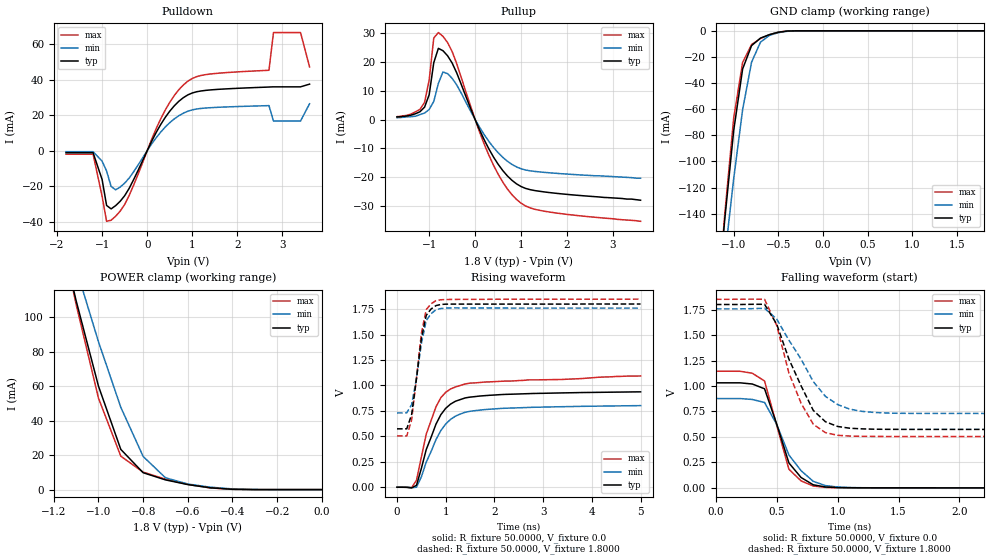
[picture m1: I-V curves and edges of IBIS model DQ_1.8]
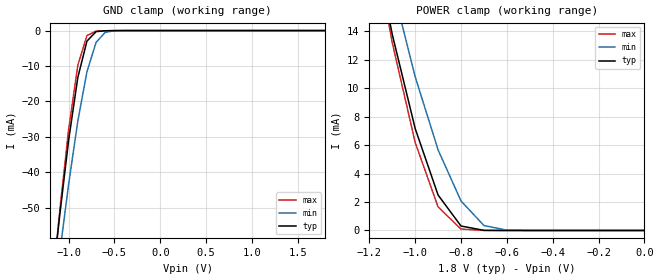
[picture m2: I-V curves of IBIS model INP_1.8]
|*** ISSI Synchronous Sram IBIS Model ***
[IBIS ver]	3.2
[File name]	is61vvps204836b119bg.ibs
[File Rev]	1.0
[Date]	May 13,2013
[Notes]
|--- Version History --------------------------------
|1.0: prelimiary
[Disclaimer]	This information is for modeling purpose only
		and is not guaranteed
[Copyright]	INTEGRATED SILICON SOLUTION, INC. 2011
[Component]	IS61VVPS204836B_119BGA
[Manufacturer]	ISSI
[Package]
| variable   typ   min   max
R_pkg		100.34m			23.84m			218.59m
L_pkg		1.3400nH		0.3700nH		3.0300nH
C_pkg		41.410pF		0.4200pF		150.38pF
[Pin]  signal_name   model_name   R_pin   L_pin   C_pin
U7   VDDQ   POWER
U6   NC   NC
U5   TDO   DQ_1.8
U4   TCK   INP_1.8
U3   TDI   INP_1.8
U2   TMS   INP_1.8
U1   VDDQ   POWER
T7   ZZ   INP_1.8
T6   A   INP_1.8
T5   A   INP_1.8
T4   A   INP_1.8
T3   A   INP_1.8
T2   A   INP_1.8
T1   NC   NC
R7   NC   NC
R6   A   INP_1.8
R5   NC   NC
R4   VDD   POWER
R3   MODE   INP_1.8
R2   A   INP_1.8
R1   NC   NC
P7   DQa   DQ_1.8
P6   DQPa   DQ_1.8
P5   VSS   GND
P4   A0   INP_1.8
P3   VSS   GND
P2   DQPd   DQ_1.8
P1   DQd   DQ_1.8
N7   DQa   DQ_1.8
N6   DQa   DQ_1.8
N5   VSS   GND
N4   A1   INP_1.8
N3   VSS   GND
N2   DQd   DQ_1.8
N1   DQd   DQ_1.8
M7   VDDQ   POWER
M6   DQa   DQ_1.8
M5   VSS   GND
M4   BWEB   INP_1.8
M3   VSS   GND
M2   DQd   DQ_1.8
M1   VDDQ   POWER
L7   DQa   DQ_1.8
L6   DQa   DQ_1.8
L5   BWaB   INP_1.8
L4   NC   NC
L3   BWdB   INP_1.8
L2   DQd   DQ_1.8
L1   DQd   DQ_1.8
K7   DQa   DQ_1.8
K6   DQa   DQ_1.8
K5   VSS   GND
K4   CLK   INP_1.8
K3   VSS   GND
K2   DQd   DQ_1.8
K1   DQd   DQ_1.8
J7   VDDQ   POWER
J6   VDD   POWER
J5   NC   NC
J4   VDD   POWER
J3   NC   NC
J2   VDD   POWER
J1   VDDQ   POWER
H7   DQb   DQ_1.8
H6   DQb   DQ_1.8
H5   VSS   GND
H4   GWB   INP_1.8
H3   VSS   GND
H2   DQc   DQ_1.8
H1   DQc   DQ_1.8
G7   DQb   DQ_1.8
G6   DQb   DQ_1.8
G5   BWbB   INP_1.8
G4   ADVB   INP_1.8
G3   BWcB   INP_1.8
G2   DQc   DQ_1.8
G1   DQc   DQ_1.8
F7   VDDQ   POWER
F6   DQb   DQ_1.8
F5   VSS   GND
F4   OEB   INP_1.8
F3   VSS   GND
F2   DQc   DQ_1.8
F1   VDDQ   POWER
E7   DQb   DQ_1.8
E6   DQb   DQ_1.8
E5   VSS   GND
E4   CEB   INP_1.8
E3   VSS   GND
E2   DQc   DQ_1.8
E1   DQc   DQ_1.8
D7   DQb   DQ_1.8
D6   DQPb   DQ_1.8
D5   VSS   GND
D4   NC   NC
D3   VSS   GND
D2   DQPc   DQ_1.8
D1   DQc   DQ_1.8
C7   NC   Nc
C6   A   INP_1.8
C5   A   INP_1.8
C4   VDD   POWER
C3   A   INP_1.8
C2   A   INP_1.8
C1   NC   NC
B7   NC   NC
B6   A   INP_1.8
B5   A   INP_1.8
B4   ADSCB   INP_1.8
B3   A   INP_1.8
B2   A   INP_1.8
B1   NC   NC
A7   VDDQ   POWER
A6   A   INP_1.8
A5   A   INP_1.8
A4   ADSPB   INP_1.8
A3   A   INP_1.8
A2   A   INP_1.8
A1   VDDQ   POWER
| Models and submodels in the file (2): DQ_1.8 (3-state), INP_1.8 (Input)
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|   Model DQ_1.8
[Model]		DQ_1.8
Model_type	3-state
Polarity   Non-Inverting
Enable   Active-Low
Vmeas = 	0.7500V
Cref = 		5.0000pF
Rref = 		50.0000
Vref = 		0.8000V
C_comp   3.8290pF   3.3420pF   4.0300pF|
[Temperature Range]	  25.0000   100.0000   0.0
[Voltage Range]   1.8000V   1.7000V   1.9000V
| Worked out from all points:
|   slope of the pulldown table from 0 to 0.27 V, typ, clamps not added: 20.1 ohm
|   slope of the pullup table from 0 to 0.27 V, typ, clamps not added: 29.1 ohm
|   GND clamp passes 1 mA (typ) near -0.49 V on its own axis
|   POWER clamp passes 1 mA (typ) near -0.49 V on its own axis
|   rising waveform, R_fixture 50.0000, V_fixture 0.0: 20-80 % time 458ps typ, 504ps min, 428ps max; typ from 0 V to 0.937 V
|   rising waveform, R_fixture 50.0000, V_fixture 1.8000: 20-80 % time 212ps typ, 215ps min, 202ps max; typ from 0.574 V to 1.8 V
|   falling waveform, R_fixture 50.0000, V_fixture 0.0: 20-80 % time 184ps typ, 232ps min, 159ps max; typ from 1.03 V to 0 V
|   falling waveform, R_fixture 50.0000, V_fixture 1.8000: 20-80 % time 261ps typ, 323ps min, 225ps max; typ from 1.8 V to 0.574 V
[Pulldown]
|Voltage	  I(typ)   I(min)   I(max)
-1.8V     -1.1mA     -531.4uA   -1.933mA
-1.2V     -1.1mA     -531.4uA   -1.933mA
-1V       -16.17mA   -5.85mA    -25.61mA
-900mV    -30.82mA   -11.44mA   -39.73mA
-800mV    -32.74mA   -20.11mA   -39.13mA
-400mV    -21.21mA   -15.41mA   -25.25mA
400mV     18.75mA    13.32mA    22.87mA
900mV     31.42mA    22.22mA    39.13mA
2.7V      35.87mA    25.41mA    45.31mA
2.8V      35.97mA    16.71mA    66.53mA
3.4V      35.97mA    16.71mA    66.53mA
3.6V      37.5mA     26.46mA    47.19mA
[Pullup]
|Voltage	  I(typ)   I(min)   I(max)
-1.7V     900uA      630uA      990uA
-1.3V     2mA        1.134mA    2.662mA
-1.1V     4.3mA      2.25mA     5.962mA
-1V       8.6mA      3.483mA    13.72mA
-900mV    19.73mA    6.273mA    28.28mA
-800mV    24.69mA    12.51mA    30.17mA
-700mV    23.88mA    16.48mA    28.87mA
-500mV    19.6mA     14.29mA    23.58mA
300mV     -10.22mA   -7.61mA    -12.41mA
900mV     -22.31mA   -16.43mA   -27.72mA
1.5V      -25.11mA   -18.32mA   -31.79mA
3.6V      -28mA      -20.34mA   -35.31mA
[GND_clamp]
|Voltage	  I(typ)   I(min)   I(max)
-1.8V     -699.5mA   -630.9mA   -769.6mA
-1.2V     -220.2mA   -237.3mA   -225.5mA
-1.1V     -144.4mA   -173.5mA   -140.5mA
-1V       -76.37mA   -113.2mA   -66.75mA
-900mV    -29.2mA    -60.35mA   -24.21mA
-800mV    -11.34mA   -23.99mA   -10.5mA
-700mV    -5.573mA   -8.7mA     -5.882mA
-600mV    -2.907mA   -3.456mA   -3.007mA
-500mV    -1.075mA   -1.407mA   -999.2uA
-400mV    -173.9uA   -365.4uA   -128uA
1.8V      2.34nA     184.5nA    2.08nA
[POWER_clamp]
|Voltage	  I(typ)   I(min)   I(max)
-1.8V     524.9mA    464.4mA    580.5mA
-1.2V     164.3mA    173.4mA    169.2mA
-1.1V     109.5mA    128.3mA    107.3mA
-1V       59.99mA    85.74mA    53.06mA
-900mV    23.31mA    47.72mA    19.37mA
-800mV    9.803mA    19.24mA    10.14mA
-700mV    5.64mA     6.854mA    6.056mA
-600mV    2.92mA     3.245mA    3.006mA
-500mV    1.061mA    1.426mA    981.4uA
-400mV    183.6uA    396.9uA    135.3uA
0V        2.34nA     17.95nA    3.205nA
[Ramp]
| variable   typ   min   max
dV/dt_r		0.5623/0.4256n   0.4811/0.4247n   0.6354/0.4100n
dV/dt_f		0.7357/0.2222n   0.6457/0.2069n   0.7931/0.2538n
R_load =	50.0000
[Rising Waveform]
R_fixture=	50.0000
V_fixture=	0.0
V_fixture_min=	0.0
V_fixture_max=	0.0
|time   V(typ)   V(min)   V(max)
0s        0V         0V         0V
300ps     -6.035mV   -4.762mV   -4.194mV
400ps     18.96mV    486.8uV    69.03mV
600ps     370.5mV    247mV      521.7mV
800ps     620mV      467.9mV    790.2mV
900ps     712.9mV    557.2mV    879.6mV
1.1ns     817.3mV    666.8mV    965.5mV
1.4ns     877.6mV    736.7mV    1.015V
1.9ns     903.3mV    766.6mV    1.035V
5ns       937.2mV    801.8mV    1.093V
[Rising Waveform]
R_fixture=	50.0000
V_fixture=	1.8000
V_fixture_min=	1.8500
V_fixture_max=	1.7500
|time   V(typ)   V(min)   V(max)
0s        573.8mV    730.3mV    504.1mV
200ps     573.9mV    730.3mV    504.2mV
300ps     713.7mV    812.3mV    659.4mV
400ps     1.067V     1.071V     1.076V
500ps     1.46V      1.412V     1.51V
600ps     1.689V     1.637V     1.745V
700ps     1.752V     1.705V     1.802V
800ps     1.784V     1.744V     1.833V
1.2ns     1.799V     1.762V     1.845V
5ns       1.8V       1.76V      1.848V
[Falling Waveform]
R_fixture=	50.0000
V_fixture=	0.0
V_fixture_min=	0.0
V_fixture_max=	0.0
|time   V(typ)   V(min)   V(max)
0s        1.031V     876.6mV    1.145V
300ps     1.019V     867.6mV    1.125V
400ps     972.5mV    838.1mV    1.049V
500ps     626.1mV    622.4mV    612.9mV
600ps     244.7mV    322.8mV    182.9mV
700ps     101.5mV    168.6mV    68.26mV
800ps     29.89mV    63.85mV    18.06mV
900ps     8.638mV    22.26mV    4.629mV
1.2ns     563.4uV    1.383mV    368.3uV
5ns       26.68uV    38.84uV    22.23uV
[Falling Waveform]
R_fixture=	50.0000
V_fixture=	1.8000
V_fixture_min=	1.8500
V_fixture_max=	1.7500
|time   V(typ)   V(min)   V(max)
0s        1.8V       1.757V     1.851V
400ps     1.802V     1.763V     1.851V
500ps     1.607V     1.657V     1.594V
600ps     1.264V     1.45V      1.127V
700ps     1.002V     1.263V     831.3mV
800ps     760.7mV    1.044V     624.3mV
900ps     649.1mV    898.2mV    542.1mV
1.1ns     585.4mV    772.7mV    508.4mV
1.4ns     574.7mV    734.9mV    504.6mV
5ns       573.8mV    730.3mV    504.2mV
|   Model INP_1.8
[Model]		INP_1.8
Model_type	Input
Polarity   Non-Inverting
Enable   Active-Low
Vinl = 		0.4000V
Vinh = 		1.6000V
C_comp   3.8290pF   3.3420pF   4.0300pF|
[Temperature Range]	  25.0000   100.0000   0.0
[Voltage Range]   1.8000V   1.7000V   1.9000V
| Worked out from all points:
|   GND clamp passes 1 mA (typ) near -0.73 V on its own axis
|   POWER clamp passes 1 mA (typ) near -0.83 V on its own axis
[GND_clamp]
|Voltage	  I(typ)   I(min)   I(max)
-1.8V     -237.3mA   -225.6mA   -256.2mA
-1.2V     -76.89mA   -84.89mA   -78.19mA
-1.1V     -52.83mA   -63.46mA   -51.66mA
-1V       -30.98mA   -43.42mA   -27.92mA
-900mV    -13.28mA   -25.61mA   -9.811mA
-800mV    -2.971mA   -11.61mA   -1.401mA
-700mV    -287uA     -3.303mA   -148.3uA
-600mV    -52.18uA   -480.7uA   -48.72uA
-500mV    -11.21uA   -45.78uA   -9.079uA
-400mV    -777.9nA   -4.481uA   -394.5nA
1.8V      1.69nA     1.724nA    1.796nA
[POWER_clamp]
|Voltage	  I(typ)   I(min)   I(max)
-1.8V     89.26mA    83.96mA    96.39mA
-1.2V     21.9mA     24.63mA    22.02mA
-1.1V     13.77mA    17.21mA    13.19mA
-1V       7.16mA     10.8mA     6.179mA
-900mV    2.488mA    5.659mA    1.649mA
-800mV    312.9uA    2.071mA    100.3uA
-700mV    9.014uA    348.8uA    1.66uA
-600mV    208.4nA    21.46uA    65.15nA
0V        1.69nA     1.088nA    2.855nA
